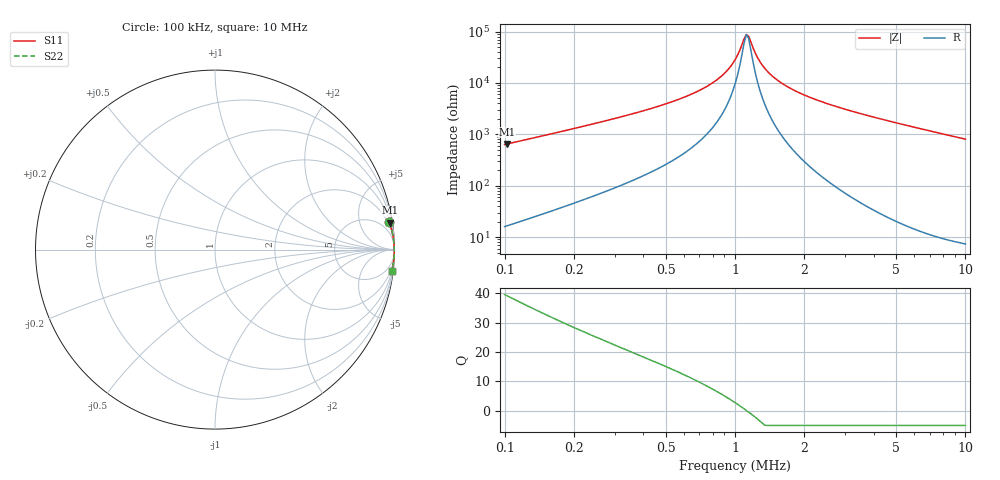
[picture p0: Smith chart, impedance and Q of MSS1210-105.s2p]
# MHz S MA R 50
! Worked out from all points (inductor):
!   203 points, 100 kHz to 10 MHz, reference 50 ohm
!   read as one part in series: L = 999 uH near 102.3 kHz
!   highest Q = 39.2 at 102.3 kHz (marker M1), where L = 1.01 mH
!   self-resonance near 1.121 MHz
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0.1  0.9839 8.9  0.1554 -79.6  0.1554 -79.6  0.9839 8.9
0.102306  0.9845 8.7  0.1519 -79.8  0.1519 -79.8  0.9845 8.7
0.1768173  0.9933 5.0  0.08725 -83.1  0.08725 -83.1  0.9933 5.0
0.2853945  0.9964 3.0  0.05205 -84.5  0.05205 -84.5  0.9964 3.0
0.7435105  0.9985 0.7  0.01213 -82.8  0.01213 -82.8  0.9985 0.7
0.8922674  0.9987 0.4  0.006742 -78.8  0.006742 -78.8  0.9987 0.4
1  0.9988 0.2  0.003558 -70.2  0.003558 -70.2  0.9988 0.2
1.095479  0.9989 0.0  0.001377 -33.8  0.001377 -33.8  0.9989 0.0
1.12074  0.9989 0.0  0.001138 -6.2  0.001138 -6.2  0.9989 0.0
1.146584  0.9989 -0.0  0.001235 25.0  0.001235 25.0  0.9989 -0.0
1.200074  0.9989 -0.1  0.002117 58.7  0.002117 58.7  0.9989 -0.1
1.256059  0.9989 -0.2  0.003284 70.8  0.003284 70.8  0.9989 -0.2
1.344971  0.9989 -0.3  0.005163 78.1  0.005163 78.1  0.9989 -0.3
1.507363  0.999 -0.5  0.008428 82.8  0.008428 82.8  0.999 -0.5
1.768173  0.999 -0.8  0.01323 85.3  0.01323 85.3  0.999 -0.8
2.07411  0.999 -1.1  0.01839 86.3  0.01839 86.3  0.999 -1.1
2.43298  0.9989 -1.4  0.02402 86.7  0.02402 86.7  0.9989 -1.4
3.424944  0.9985 -2.2  0.03834 86.7  0.03834 86.7  0.9985 -2.2
5.162633  0.9974 -3.5  0.06163 85.8  0.06163 85.8  0.9974 -3.5
6.787083  0.9958 -4.7  0.08259 84.7  0.08259 84.7  0.9958 -4.7
8.524974  0.9936 -6.0  0.1046 83.5  0.1046 83.5  0.9936 -6.0
10  0.9913 -7.1  0.123 82.4  0.123 82.4  0.9913 -7.1
